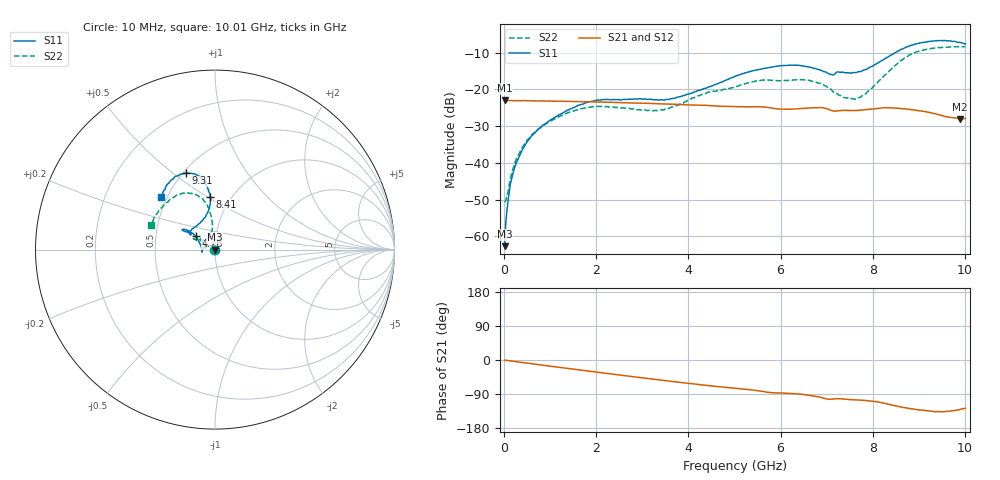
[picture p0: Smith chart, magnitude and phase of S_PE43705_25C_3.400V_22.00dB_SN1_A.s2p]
! Device ID: PE43705
! Serial: 1
! Insertion: A
! Impedance: 50 ohm
! Temp: 25C
! VDD: 3.400V
! Attenuation Step: 22.00dB
#  Hz  S  RI  R  50
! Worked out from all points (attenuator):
!   401 points, 10 MHz to 10.01 GHz, reference 50 ohm
!   highest |S21| = -23.02 dB at 10 MHz (marker M1); lowest = -28.0 dB at 9.885 GHz (marker M2)
!   lowest |S11| = -62.7 dB at 10 MHz (marker M3), VSWR 1.00, Z = 49.9 + j0.0417 ohm
!   |S11| at or under -10 dB: start of sweep to 8.485 GHz
!   |S22| runs from -50.7 to -8.3 dB; largest |S21 - S12| = 0.00077
!   S11 on the Smith chart (normalised r, x): 10 MHz: 1.00, +0.00; 4.76 GHz: 0.80, +0.12; 8.41 GHz: 0.80, +0.52; 9.31 GHz: 0.52, +0.56; 10.01 GHz: 0.46, +0.33
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1e7  -0.000604 0.000417  0.0707 -0.000272  0.0707 -0.000234  -0.00288 0.0005
8.5e7  -0.000388 0.00302  0.0704 -0.00188  0.0705 -0.00181  -0.00227 0.00341
1.6e8  -0.000816 0.00598  0.0704 -0.00337  0.0703 -0.00334  -0.00252 0.00657
2.6e8  -0.00213 0.00966  0.07 -0.0054  0.07 -0.0054  -0.00364 0.0105
4.35e8  -0.00593 0.0155  0.0698 -0.00893  0.0696 -0.00879  -0.00668 0.0165
8.6e8  -0.0242 0.0225  0.0675 -0.0169  0.0675 -0.0169  -0.0217 0.0244
1.685e9  -0.0618 0.00975  0.0606 -0.0308  0.0607 -0.0308  -0.0521 0.0167
2.16e9  -0.0726 -0.00492  0.0554 -0.0378  0.0554 -0.0378  -0.0578 0.00699
3.36e9  -0.0716 -0.00416  0.0387 -0.0506  0.0388 -0.0505  -0.05 0.0128
4.76e9  -0.106 0.0737  0.0186 -0.0558  0.0187 -0.0559  -0.0812 0.0583
5.01e9  -0.1219 0.0887  0.0153 -0.0562  0.0156 -0.0562  -0.089 0.0633
5.985e9  -0.1767 0.1131  0.00275 -0.054  0.00285 -0.0538  -0.11 0.0713
6.685e9  -0.1684 0.1009  -0.00441 -0.0559  -0.00432 -0.0557  -0.1145 0.0589
7.11e9  -0.1336 0.086  -0.012 -0.05  -0.0118 -0.0501  -0.0815 0.0537
7.585e9  -0.0938 0.1413  -0.0133 -0.0497  -0.0134 -0.0497  -0.0402 0.0626
7.885e9  -0.0522 0.1837  -0.016 -0.0508  -0.0156 -0.0507  -0.0218 0.0905
8.36e9  -0.0249 0.2833  -0.0258 -0.0503  -0.0258 -0.0501  -0.0197 0.1788
8.41e9  -0.028 0.2951  -0.0268 -0.049  -0.0269 -0.0492  -0.023 0.1894
8.835e9  -0.0712 0.3911  -0.0333 -0.0412  -0.0329 -0.0415  -0.0805 0.2902
9.31e9  -0.1628 0.4262  -0.0336 -0.033  -0.0337 -0.033  -0.1878 0.3118
9.885e9  -0.2839 0.3318  -0.026 -0.03  -0.026 -0.0299  -0.3342 0.1867
1.001e10  -0.3003 0.2916  -0.0245 -0.032  -0.0247 -0.0315  -0.3584 0.1359
